(* Logix 5000 DataType export Set_Parameter; software revision 32.01 *)

TYPE Set_Parameter :
STRUCT
   Address : SINT;   // 1-31=Address 1-31, 32-62=Address 1B-31B
   Parameter : SINT;   // Parameter to Set
END_STRUCT
END_TYPE
